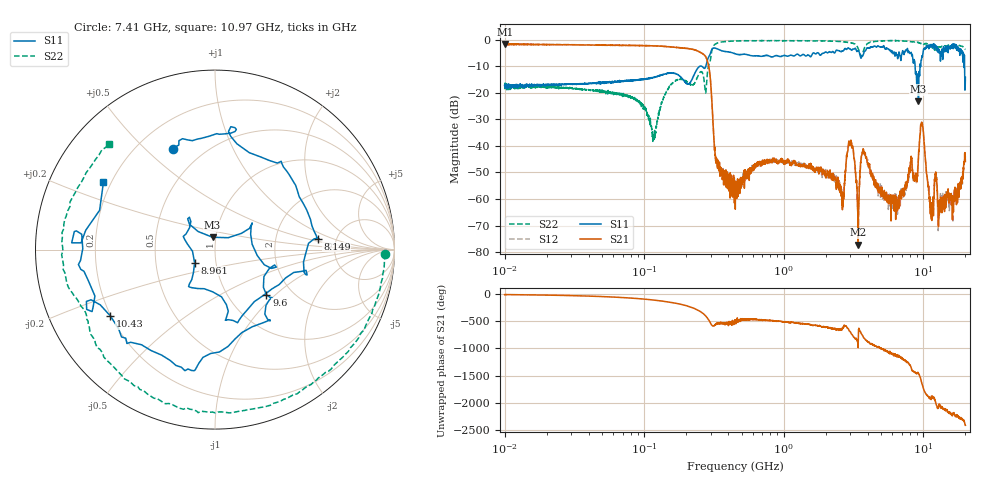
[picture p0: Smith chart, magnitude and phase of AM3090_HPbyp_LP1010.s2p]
# Hz S DB R 50
!freq MagS11 AngS11 MagS21 AngS21 MagS12 AngS12 MagS22 AngS22
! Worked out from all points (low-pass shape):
!   3201 points, 10 MHz to 20 GHz, reference 50 ohm
!   highest |S21| = -1.49 dB at 10.05 MHz (marker M1); lowest = -77.3 dB at 3.416 GHz (marker M2)
!   |S21| within 3 dB of the highest: start of sweep to 247.4 MHz
!   lowest |S11| = -23.1 dB at 9.22 GHz (marker M3), VSWR 1.15, Z = 48.2 + j6.66 ohm
!   |S11| at or under -10 dB: start of sweep to 248.6 MHz; 8.728 GHz to 9.457 GHz (728.4 MHz wide, 8.01 % of centre); 19.73 GHz to end of sweep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
!   |S22| runs from -38.3 to -0.2 dB; largest |S21 - S12| = 0.041
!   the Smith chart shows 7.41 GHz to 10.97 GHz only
!   S11 on the Smith chart (normalised r, x): 7.41 GHz: 0.34, +0.61; 8.149 GHz: 3.57, +0.65; 8.961 GHz: 0.79, -0.12; 9.6 GHz: 1.49, -0.88; 10.43 GHz: 0.20, -0.28; 10.97 GHz: 0.17, +0.27
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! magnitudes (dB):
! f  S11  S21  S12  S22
! 10 MHz  -17.0  -1.8  -1.7  -17.2
! 10.05 MHz  -17.8  -1.5  -1.7  -18.0
! 35.55 MHz  -16.6  -1.9  -1.9  -18.7
! 126.1 MHz  -13.7  -2.3  -2.3  -29.5
! 275.5 MHz  -10.2  -6.4  -6.2  -20.0
! 332.3 MHz  -3.3  -46.1  -46.8  -1.3
! 447.2 MHz  -5.2  -53.5  -55.6  -0.4
! 1.59 GHz  -5.7  -47.7  -47.4  -0.3
! 2.606 GHz  -4.2  -57.3  -60.1  -0.6
! 3.012 GHz  -3.5  -38.0  -37.9  -1.1
! 3.416 GHz  -4.1  -77.3  -69.7  -3.3
! 3.748 GHz  -4.8  -42.2  -42.5  -3.5
! 5.639 GHz  -3.6  -61.3  -60.1  -0.3
! 7.41 GHz  -4.3  -54.9  -55.1  -0.5
! 8.149 GHz  -4.8  -44.9  -46.2  -0.7
! 8.961 GHz  -17.4  -51.1  -51.9  -0.9
! 9.22 GHz  -23.1  -44.2  -44.4  -1.0
! 9.6 GHz  -8.4  -31.8  -32.3  -1.4
! 10.43 GHz  -3.2  -47.1  -46.9  -1.4
! 10.97 GHz  -2.8  -57.5  -57.4  -1.6
! 15.92 GHz  -2.5  -62.1  -62.2  -1.8
! 20 GHz  -14.1  -45.9  -43.7  -3.6
